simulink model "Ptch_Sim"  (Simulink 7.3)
settings: Solver=ode45  StartTime=0.0  StopTime=250  RelTol=1e-3
InitFcn:
  | init
StopFcn:
  | Pl
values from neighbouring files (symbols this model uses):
  Aac = [    [actuator.m]
  Bac = [    [actuator.m]
  Cac = [    [actuator.m]
  Cza = -0.343    [init.m]
  d2r = pi/180    (= 0.0174532925199)    [init.m]    (also in run.m; LQR_Des.m)
  Dac = [    [actuator.m]
  Kc = [12.6, 3.15, -0.3, 0.37]*0.127    [init.m]
  Mass = 9580    [init.m]
  Qbar = 228    [init.m]
  r2d = 1/d2r    (= 57.2957795131)    [init.m]    (also in Pl.m; run.m; LQR_Des.m)
  Sref = 47.3    [init.m]
  Thr = 363305    [init.m]
undefined symbols (not defined in the file or in its folder): Avf, Bvf, Cvf, Dvf

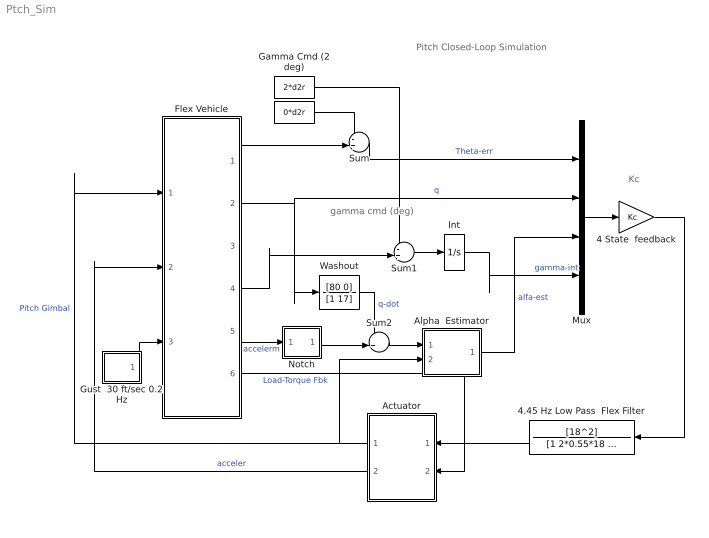
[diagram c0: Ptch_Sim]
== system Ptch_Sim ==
  note: Pitch Closed-Loop Simulation
  note: gamma cmd (deg)
  note: Kc
  " " : Constant  Value=0*d2r  OutDataType=sfix(16)  OutScaling=2^0
  4 State  feedback : Gain  Gain=Kc  Multiplication=Matrix(K*u)  ParameterDataType=sfix(16)  ParameterScaling=2^0  OutDataType=sfix(16)  OutScaling=2^0
  4.45 Hz Low Pass  Flex Filter : TransferFcn  Numerator=[18^2]  Denominator="[1 2*0.55*18  18^2]"
  Actuator : Subsystem
  Alpha  Estimator : Subsystem
  Flex Vehicle : Subsystem
  Gamma Cmd (2 deg) : Constant  Value=2*d2r  OutDataType=sfix(16)  OutScaling=2^0
  Gust  30 ft/sec 0.2 Hz : Subsystem
  Int : Integrator
  Mux : Mux
  Notch : Subsystem
  Sum : Sum  Inputs=-+|  OutDataType=sfix(16)  OutScaling=2^0
  Sum1 : Sum  Inputs=-+|  OutDataType=sfix(16)  OutScaling=2^0
  Sum2 : Sum  Inputs=++|  OutDataType=sfix(16)  OutScaling=2^0
  Washout : TransferFcn  Numerator=[80 0]  Denominator=[1 17]
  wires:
  Flex Vehicle/2(q-flex) -> Mux/2, Washout/1  "q"
  Int/1 -> Mux/4  "gamma-int"
  Mux/1 -> 4 State  feedback/1
  Flex Vehicle/1(theta) -> Sum/2
  Sum/1 -> Mux/1  "Theta-err"
  Flex Vehicle/4(gama) -> Sum1/2
  Sum1/1 -> Int/1
  4 State  feedback/1 -> 4.45 Hz Low Pass  Flex Filter/1
  Alpha  Estimator/1(alphat) -> Mux/3  "alfa-est"
  Actuator/1(Dy) -> Alpha  Estimator/2(delta), Flex Vehicle/1(Dy)  "Pitch Gimbal"
  Gust  30 ft/sec 0.2 Hz/1(Vgust) -> Flex Vehicle/3(Gust)
  " "/1 -> Sum/1
  Sum2/1 -> Alpha  Estimator/1(Zdd)
  Washout/1 -> Sum2/1  "q-dot"
  Notch/1(Ou) -> Sum2/2
  Flex Vehicle/5(Zdd-flex) -> Notch/1(In)  "accelerm"
  Gamma Cmd (2 deg)/1 -> Sum1/1
  4.45 Hz Low Pass  Flex Filter/1 -> Actuator/1(Dyc)
  Flex Vehicle/6(TLy) -> Actuator/2(TLy)  "Load-Torque Fbk"
  Actuator/2(Dy_dd) -> Flex Vehicle/2(Dy_dd)  "acceler"

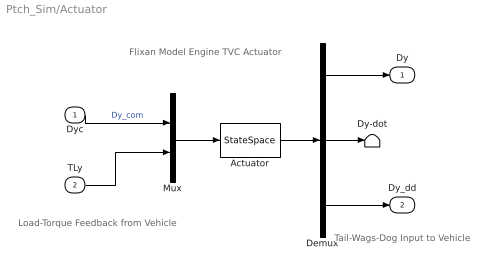
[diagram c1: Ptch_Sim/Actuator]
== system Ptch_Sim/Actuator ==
  note: Tail-Wags-Dog Input to Vehicle
  note: Load-Torque Feedback from Vehicle
  note: Flixan Model Engine TVC Actuator
  Dyc : Inport  OutDataType=sfix(16)  OutScaling=2^0
  TLy : Inport  Port=2  OutDataType=sfix(16)  OutScaling=2^0
  Actuator : StateSpace  A=Aac  B=Bac  C=Cac  D=Dac
  Demux : Demux  Outputs=3
  Dy-dot : Terminator
  Mux : Mux  Inputs=2
  Dy : Outport  OutDataType=sfix(16)  OutScaling=2^0
  Dy_dd : Outport  Port=2  OutDataType=sfix(16)  OutScaling=2^0
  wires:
  Mux/1 -> Actuator/1
  Actuator/1 -> Demux/1
  Demux/2 -> Dy-dot/1
  Dyc/1 -> Mux/1  "Dy_com"
  Demux/1 -> Dy/1
  Demux/3 -> Dy_dd/1
  TLy/1 -> Mux/2

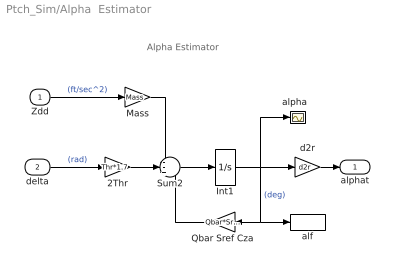
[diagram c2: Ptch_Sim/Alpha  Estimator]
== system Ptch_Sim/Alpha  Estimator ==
  note: Alpha Estimator
  Zdd : Inport  OutDataType=sfix(16)  OutScaling=2^0
  delta : Inport  Port=2  OutDataType=sfix(16)  OutScaling=2^0
  2Thr : Gain  Gain=Thr*1.7  ParameterDataType=sfix(16)  ParameterScaling=2^0  OutDataType=sfix(16)  OutScaling=2^0
  Int1 : Integrator
  Mass : Gain  Gain=Mass  ParameterDataType=sfix(16)  ParameterScaling=2^0  OutDataType=sfix(16)  OutScaling=2^0
  Qbar Sref Cza : Gain  Gain=Qbar*Sref*Cza  ParameterDataType=sfix(16)  ParameterScaling=2^0  OutDataType=sfix(16)  OutScaling=2^0
  Sum2 : Sum  Inputs=--+  OutDataType=sfix(16)  OutScaling=2^0
  alf : ToWorkspace  VariableName=alphat  SampleTime=-1  SaveFormat=Array
  "alpha  " : Scope
  d2r : Gain  Gain=d2r  ParameterDataType=sfix(16)  ParameterScaling=2^0  OutDataType=sfix(16)  OutScaling=2^0
  alphat : Outport  OutDataType=sfix(16)  OutScaling=2^0
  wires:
  Sum2/1 -> Int1/1
  2Thr/1 -> Sum2/2
  Int1/1 -> d2r/1, "alpha  "/1, Qbar Sref Cza/1, alf/1  "(deg)"
  Qbar Sref Cza/1 -> Sum2/3
  delta/1 -> 2Thr/1  "(rad)"
  Zdd/1 -> Mass/1  "(ft/sec^2)"
  Mass/1 -> Sum2/1
  d2r/1 -> alphat/1

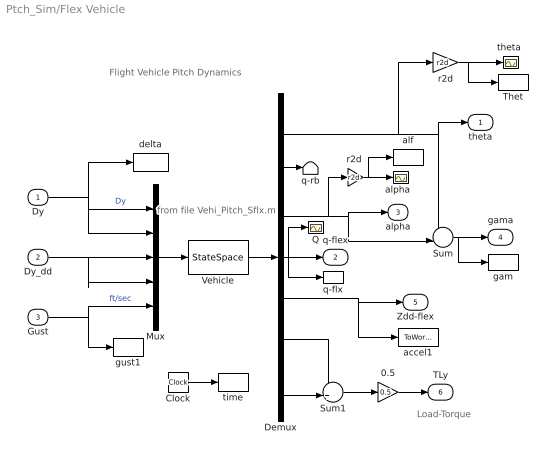
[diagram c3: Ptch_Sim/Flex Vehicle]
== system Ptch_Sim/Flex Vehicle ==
  note: Flight Vehicle Pitch Dynamics
  note: from file Vehi_Pitch_Sflx.m
  note: Load-Torque
  Dy : Inport  OutDataType=sfix(16)  OutScaling=2^0
  Dy_dd : Inport  Port=2  OutDataType=sfix(16)  OutScaling=2^0
  Gust : Inport  Port=3  OutDataType=sfix(16)  OutScaling=2^0
  0.5 : Gain  Gain=0.5  ParameterDataType=sfix(16)  ParameterScaling=2^0  OutDataType=sfix(16)  OutScaling=2^0
  Clock : Clock
  Demux : Demux  Outputs=7
  Mux : Mux  Inputs=5
  Q : Scope
  Sum : Sum  Inputs=+-|  OutDataType=sfix(16)  OutScaling=2^0
  Sum1 : Sum  Inputs=++|  OutDataType=sfix(16)  OutScaling=2^0
  Thet : ToWorkspace  VariableName=theta  SampleTime=-1  SaveFormat=Array
  Vehicle : StateSpace  A=Avf  B=Bvf  C=Cvf  D=Dvf
  accel1 : ToWorkspace  VariableName=accel  SampleTime=-1  SaveFormat=Array
  alf : ToWorkspace  VariableName=alpha  SampleTime=-1  SaveFormat=Array
  "alpha  " : Scope
  delta : ToWorkspace  VariableName=delta  SampleTime=-1  SaveFormat=Array
  gam : ToWorkspace  VariableName=gama  SampleTime=-1  SaveFormat=Array
  gust1 : ToWorkspace  VariableName=Gust  SampleTime=-1  SaveFormat=Array
  q-flx : ToWorkspace  VariableName=q  SampleTime=-1  SaveFormat=Array
  q-rb : Terminator
  r2d : Gain  Gain=r2d  ParameterDataType=sfix(16)  ParameterScaling=2^0  OutDataType=sfix(16)  OutScaling=2^0
  "r2d " : Gain  Gain=r2d  ParameterDataType=sfix(16)  ParameterScaling=2^0  OutDataType=sfix(16)  OutScaling=2^0
  "theta " : Scope
  time : ToWorkspace  VariableName=time  SampleTime=-1  SaveFormat=Array
  theta : Outport  OutDataType=sfix(16)  OutScaling=2^0
  q-flex : Outport  Port=2  OutDataType=sfix(16)  OutScaling=2^0
  alpha : Outport  Port=3  OutDataType=sfix(16)  OutScaling=2^0
  gama : Outport  Port=4  OutDataType=sfix(16)  OutScaling=2^0
  Zdd-flex : Outport  Port=5  OutDataType=sfix(16)  OutScaling=2^0
  TLy : Outport  Port=6  OutDataType=sfix(16)  OutScaling=2^0
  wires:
  Mux/1 -> Vehicle/1
  Vehicle/1 -> Demux/1
  Dy/1 -> Mux/1, Mux/2, delta/1  "Dy"
  Gust/1 -> Mux/5, gust1/1  "ft/sec"
  Dy_dd/1 -> Mux/3, Mux/4
  Demux/1 -> theta/1, Sum/1, r2d/1
  Demux/3 -> Sum/2, alpha/1, "r2d "/1
  Demux/5 -> Zdd-flex/1, accel1/1
  Demux/7 -> Sum1/2
  Demux/6 -> Sum1/1
  Sum/1 -> gama/1, gam/1
  Demux/4 -> q-flex/1, q-flx/1, Q/1
  Demux/2 -> q-rb/1
  Clock/1 -> time/1
  r2d/1 -> "theta "/1, Thet/1
  "r2d "/1 -> "alpha  "/1, alf/1
  0.5/1 -> TLy/1
  Sum1/1 -> 0.5/1

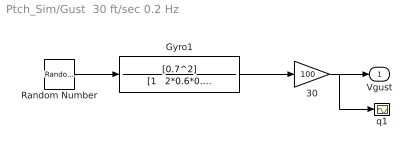
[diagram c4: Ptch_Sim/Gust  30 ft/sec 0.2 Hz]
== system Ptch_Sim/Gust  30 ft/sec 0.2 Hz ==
  30 : Gain  Gain=100  ParameterDataType=sfix(16)  ParameterScaling=2^0  OutDataType=sfix(16)  OutScaling=2^0
  Gyro1 : TransferFcn  Numerator=[0.7^2]  Denominator="[1   2*0.6*0.7   0.7^2]"
  Random Number : RandomNumber  Seed=-2  SampleTime=0
  q1 : Scope
  Vgust : Outport  OutDataType=sfix(16)  OutScaling=2^0
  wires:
  30/1 -> q1/1, Vgust/1
  Gyro1/1 -> 30/1
  Random Number/1 -> Gyro1/1

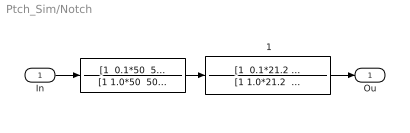
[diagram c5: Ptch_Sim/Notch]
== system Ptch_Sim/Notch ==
  In : Inport
  " " : TransferFcn  Numerator="[1  0.1*50  50^2]"  Denominator="[1 1.0*50  50^2]"
  " 1" : TransferFcn  Numerator="[1  0.1*21.2  21.2^2]"  Denominator="[1 1.0*21.2  21.2^2]"
  Ou : Outport
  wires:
  " 1"/1 -> Ou/1
  In/1 -> " "/1
  " "/1 -> " 1"/1
